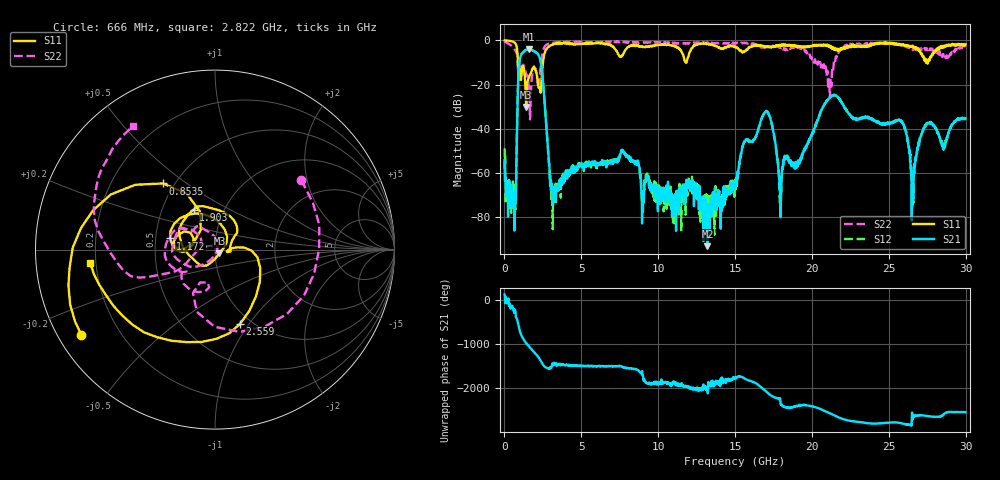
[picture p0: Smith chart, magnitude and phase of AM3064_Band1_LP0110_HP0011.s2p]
# Hz S DB R 50.0
!freq dBS11 angS11 dBS21 angS21 dBS12 angS12 dBS22 angS22
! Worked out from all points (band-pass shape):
!   1600 points, 10 MHz to 29.98 GHz, reference 50 ohm
!   highest |S21| = -4.05 dB at 1.584 GHz (marker M1); lowest = -93.0 dB at 13.21 GHz (marker M2)
!   |S21| within 3 dB of the highest: 1.054 GHz to 2.248 GHz (1.195 GHz wide, 72.4 % of centre)
!   lowest |S11| = -30.1 dB at 1.416 GHz (marker M3), VSWR 1.06, Z = 52.5 - j2.05 ohm
!   |S11| at or under -10 dB: 876.6 MHz to 2.507 GHz (1.631 GHz wide, 96.4 % of centre); 11.80848 GHz to 11.83392 GHz (25.44 MHz wide, 0.215 % of centre); 27.50984 GHz to 27.55297 GHz (43.12 MHz wide, 0.157 % of centre)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
!   |S22| runs from -35.7 to -0.4 dB; largest |S21 - S12| = 0.0075
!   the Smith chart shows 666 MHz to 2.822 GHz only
!   S11 on the Smith chart (normalised r, x): 666 MHz: 0.07, -0.29; 853.5 MHz: 0.43, +0.41; 1.172 GHz: 0.60, +0.08; 1.903 GHz: 0.72, +0.34; 2.559 GHz: 0.89, -0.91; 2.822 GHz: 0.18, -0.05
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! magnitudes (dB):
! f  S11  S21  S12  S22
! 10 MHz  0.0  -54.1  -48.9  -0.4
! 666 MHz  -1.1  -69.0  -65.6  -4.2
! 853.5 MHz  -6.6  -27.9  -27.9  -8.8
! 1.172 GHz  -11.8  -5.6  -5.6  -11.6
! 1.416 GHz  -30.1  -4.2  -4.2  -15.7
! 1.584 GHz  -16.7  -4.0  -4.1  -21.0
! 1.903 GHz  -11.9  -4.8  -4.8  -12.4
! 2.559 GHz  -7.2  -23.3  -23.3  -3.6
! 2.822 GHz  -3.1  -47.9  -47.7  -1.6
! 3.196 GHz  -1.6  -69.5  -66.2  -1.1
! 5.015 GHz  -1.5  -55.4  -56.4  -0.6
! 10 GHz  -2.1  -66.7  -68.1  -0.9
! 13.21 GHz  -1.4  -93.0  -71.2  -1.0
! 15 GHz  -3.0  -63.4  -63.0  -1.5
! 16.97 GHz  -2.7  -32.3  -32.4  -3.1
! 17.95 GHz  -2.4  -79.9  -76.8  -2.8
! 19.99 GHz  -2.7  -42.6  -42.5  -8.3
! 21.42 GHz  -3.8  -24.7  -24.6  -10.6
! 25 GHz  -1.0  -37.4  -37.9  -1.2
! 26.55 GHz  -2.3  -67.9  -62.6  -4.4
! 27.43 GHz  -10.2  -38.1  -38.3  -3.9
! 29.98 GHz  -1.7  -35.1  -35.3  -3.0
